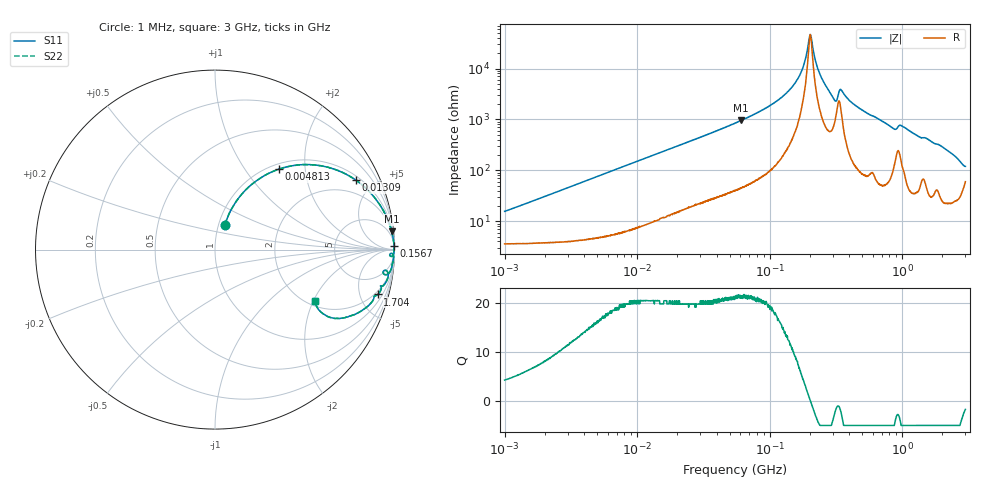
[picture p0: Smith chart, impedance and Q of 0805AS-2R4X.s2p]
!s-Parameter Generated by FASTRON Sdn. Bhd.
!FASTRON P/N : 0805AS-2R4X
!Keysight Technologies: E4991B_MY54100416_A.01.15
!Date: Mon Jun 15 12:57:58 2026
!Version  :Rev01  Mon Jun 15 12:57:58 2026
!Data & Calibration Information:
!Freq  S11  S21  S12  S22
!PortZ  Port1:50+j0  Port2:50+j0
!When reading reference impedance value at option line is always used.
! Remarks : This data is being provided solely for informational purposes.
# Hz S dB R 50
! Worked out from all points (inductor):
!   1601 points, 1 MHz to 3 GHz, reference 50 ohm
!   read as one part in series: L = 2.41 uH near 1.041 MHz
!   highest Q = 21.4 at 60.84 MHz (marker M1), where L = 2.5 uH
!   self-resonance near 202.2 MHz
!   S11 on the Smith chart (normalised r, x): 1 MHz: 1.07, +0.31; 4.813 MHz: 1.09, +1.45; 13.09 MHz: 1.19, +3.92; 156.7 MHz: open; 1.704 GHz: 1.63, -7.03; 3 GHz: 2.20, -2.07
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1000000  -16.50 68.4  -0.40 -8.3  -0.40 -8.3  -16.50 68.4
3804036  -6.30 56.9  -1.51 -28.9  -1.51 -28.9  -6.30 56.9
4812659  -4.86 51.6  -2.10 -34.8  -2.10 -34.8  -4.86 51.6
1.309258e7  -1.17 26.4  -7.03 -60.8  -7.03 -60.8  -1.17 26.4
1.447069e7  -1.00 24.3  -7.71 -62.9  -7.71 -62.9  -1.00 24.3
5.504702e7  -0.11 6.7  -18.70 -80.6  -18.70 -80.6  -0.11 6.7
6.084121e7  -0.09 6.0  -19.70 -81.3  -19.70 -81.3  -0.09 6.0
1.103592e8  -0.03 2.6  -26.90 -84.2  -26.90 -84.2  -0.03 2.6
1.566509e8  -0.02 1.1  -34.50 -82.6  -34.50 -82.6  -0.02 1.1
1.793119e8  -0.02 0.5  -40.80 -76.3  -40.80 -76.3  -0.02 0.5
1.991803e8  -0.02 0.1  -52.10 -29.9  -52.10 -29.9  -0.02 0.1
2.083556e8  -0.02 -0.1  -50.60 43.6  -50.60 43.6  -0.02 -0.1
2.223601e8  -0.02 -0.4  -42.80 71.5  -42.80 71.5  -0.02 -0.4
2.373059e8  -0.02 -0.7  -38.30 77.4  -38.30 77.4  -0.02 -0.7
3.062963e8  -0.12 -2.2  -28.00 69.3  -28.00 69.3  -0.12 -2.2
3.48855e8  -0.08 -1.4  -31.50 69.0  -31.50 69.0  -0.08 -1.4
4.593788e8  -0.04 -3.2  -25.00 83.3  -25.00 83.3  -0.04 -3.2
7.925923e8  -0.16 -7.3  -17.90 78.2  -17.90 78.2  -0.16 -7.3
9.878038e8  -0.28 -7.3  -17.80 72.1  -17.80 72.1  -0.28 -7.3
1.704314e9  -0.53 -15.4  -11.50 69.5  -11.50 69.5  -0.53 -15.4
2.634014e9  -1.90 -28.4  -6.35 52.5  -6.35 52.5  -1.90 -28.4
3e9  -4.05 -27.0  -5.59 32.9  -5.59 32.9  -4.05 -27.0
